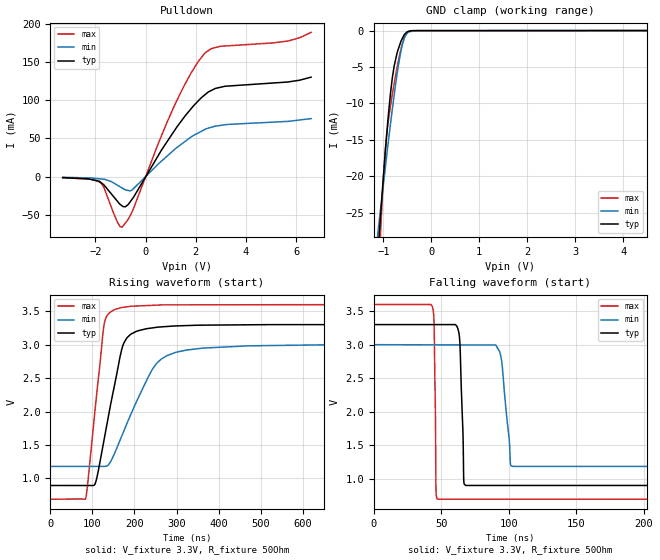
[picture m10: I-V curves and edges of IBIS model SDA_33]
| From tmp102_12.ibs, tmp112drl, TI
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|   SDA_33  3.3V digital I/O open drain Model
[Model] SDA_33
Model_type   I/O_open_drain
| Signals   SDA(6)
Polarity   Non-Inverting
Enable   Active-Low
Vinl = 0.99
Vinh = 2.31
Vmeas = 1.65
Vref = 1.65
Cref = 15pF
Rref = 50
|   typ   min   max
|   (nom PVT)   (Fast PVT)   (slow PVT)
|Average
|C_comp   6.0655910e-11  3.8241870e-11  9.0001040e-11
| Where   nom PVT is  Nominal Process, 3.3V, 27C
|   Fast PVT is Strong Process, 3.6V, 125C
|   Slow PVT is Weak Process, 3.0V, -40C
|   output high
C_comp   1.3048590e-12  1.3040560e-12  1.3136780e-12
| Where   nom PVT is  Nominal Process, 1.5V, 27C
|   Fast PVT is Strong Process, 1.6V, -40C
|   Slow PVT is Weak Process, 1.4V, 125C
[Voltage Range]   3.3   3   3.6
[Temperature Range]   27   125   -40
|Ambient Temperature   27   125   -40
[Pullup Reference]   3.3   3   3.6
[Pulldown Reference]   0   0   0
[Power Clamp Reference]   3.3   3   3.6
[GND Clamp Reference]   0   0   0
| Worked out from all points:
|   slope of the pulldown table from 0 to 0.495 V, typ, clamps not added: 18 ohm
|   GND clamp passes 1 mA (typ) near -0.60 V on its own axis
|   falling waveform, V_fixture 3.3V, R_fixture 50Ohm: 20-80 % time 2.17ns typ, 5.11ns min, 994ps max; typ from 3.3 V to 0.895 V
|   rising waveform, V_fixture 3.3V, R_fixture 50Ohm: 20-80 % time 43.9ns typ, 79ns min, 28.3ns max; typ from 0.895 V to 3.3 V
[Pulldown]
|   Voltage   I(typ)   I(min)   I(max)
-3.3V     -1.306mA   -848.7uA   -1.411mA
-1.794V   -7.28mA    -2.991mA   -8.045mA
-1.115V   -32.51mA   -11.34mA   -59.98mA
-936.2mV  -38.21mA   -14.8mA    -66.09mA
-799.9mV  -39.31mA   -17.38mA   -60.5mA
-529.9mV  -29.19mA   -17.3mA    -45.41mA
1.172V    61.35mA    36.14mA    94.61mA
1.819V    89.14mA    52.05mA    136.1mA
2.351V    106.8mA    61.55mA    161.3mA
3.155V    118.2mA    67.81mA    170.9mA
5.669V    123.8mA    72.31mA    177.4mA
6.59V     130.2mA    75.92mA    188.8mA
[GND Clamp]
|   Voltage   I(typ)   I(min)   I(max)
-3.3V     -253.2mA   -163mA     -417mA
-1.109V   -30.01mA   -27.42mA   -35.08mA
-1.054V   -24.92mA   -24.23mA   -27.05mA
-996.5mV  -19.82mA   -20.95mA   -19.91mA
-953.3mV  -16.1mA    -18.46mA   -15.87mA
-898.7mV  -11.79mA   -15.37mA   -12.5mA
-812.6mV  -6.459mA   -10.77mA   -8.709mA
-722.4mV  -3.307mA   -6.351mA   -5.349mA
-646.3mV  -1.721mA   -3.221mA   -2.913mA
-561.3mV  -543uA     -1.011mA   -954.1uA
-499.9mV  -161.8uA   -350.2uA   -263.7uA
6.59V     0A         0A         0A
[POWER Clamp]
|   SCR cell for ESD function. Effects occurr above VDD x 2
|   Voltage   I(typ)   I(min)   I(max)
-3.3V     0A         0A         0A
0V        0A         0A         0A
6.6V      0A         0A         0A
[Ramp]
R_load = 50
|   typ   min   max
dV/dt_r   1.44306/4.37551e-008   1.09207/7.89458e-008   1.74665/2.81923e-008
dV/dt_f   1.44306/2.16526e-009   1.09207/5.12036e-009   1.74665/9.92954e-010
[Falling Waveform]
V_fixture = 3.3V
V_fixture_min = 3V
V_fixture_max = 3.6V
R_fixture = 50Ohm
C_fixture = 0F
|   Time   V(typ)   V(min)   V(max)
0s        3.3V       3V         3.6V
43.38ns   3.3V       2.997V     3.567V
44.69ns   3.3V       2.997V     3.258V
46.08ns   3.3V       2.997V     813.5mV
47.58ns   3.3V       2.997V     690.6mV
63.06ns   3.172V     2.996V     690.6mV
68.11ns   896.2mV    2.996V     690.6mV
93.09ns   896.1mV    2.9V       690.5mV
102.8ns   896.1mV    1.181V     690.5mV
985.8ns   894.9mV    1.18V      688.9mV
[Rising Waveform]
V_fixture = 3.3V
V_fixture_min = 3V
V_fixture_max = 3.6V
R_fixture = 50Ohm
C_fixture = 0F
|   Time   V(typ)   V(min)   V(max)
0s        894.9mV    1.18V      688.9mV
84.05ns   894.4mV    1.18V      700.7mV
106.4ns   917.5mV    1.18V      2.027V
127ns     1.552V     1.18V      3.264V
151.1ns   2.349V     1.353V     3.519V
169.7ns   2.931V     1.633V     3.555V
182.6ns   3.106V     1.829V     3.566V
244.8ns   3.252V     2.655V     3.588V
297.1ns   3.28V      2.883V     3.595V
985.8ns   3.3V       3V         3.6V
